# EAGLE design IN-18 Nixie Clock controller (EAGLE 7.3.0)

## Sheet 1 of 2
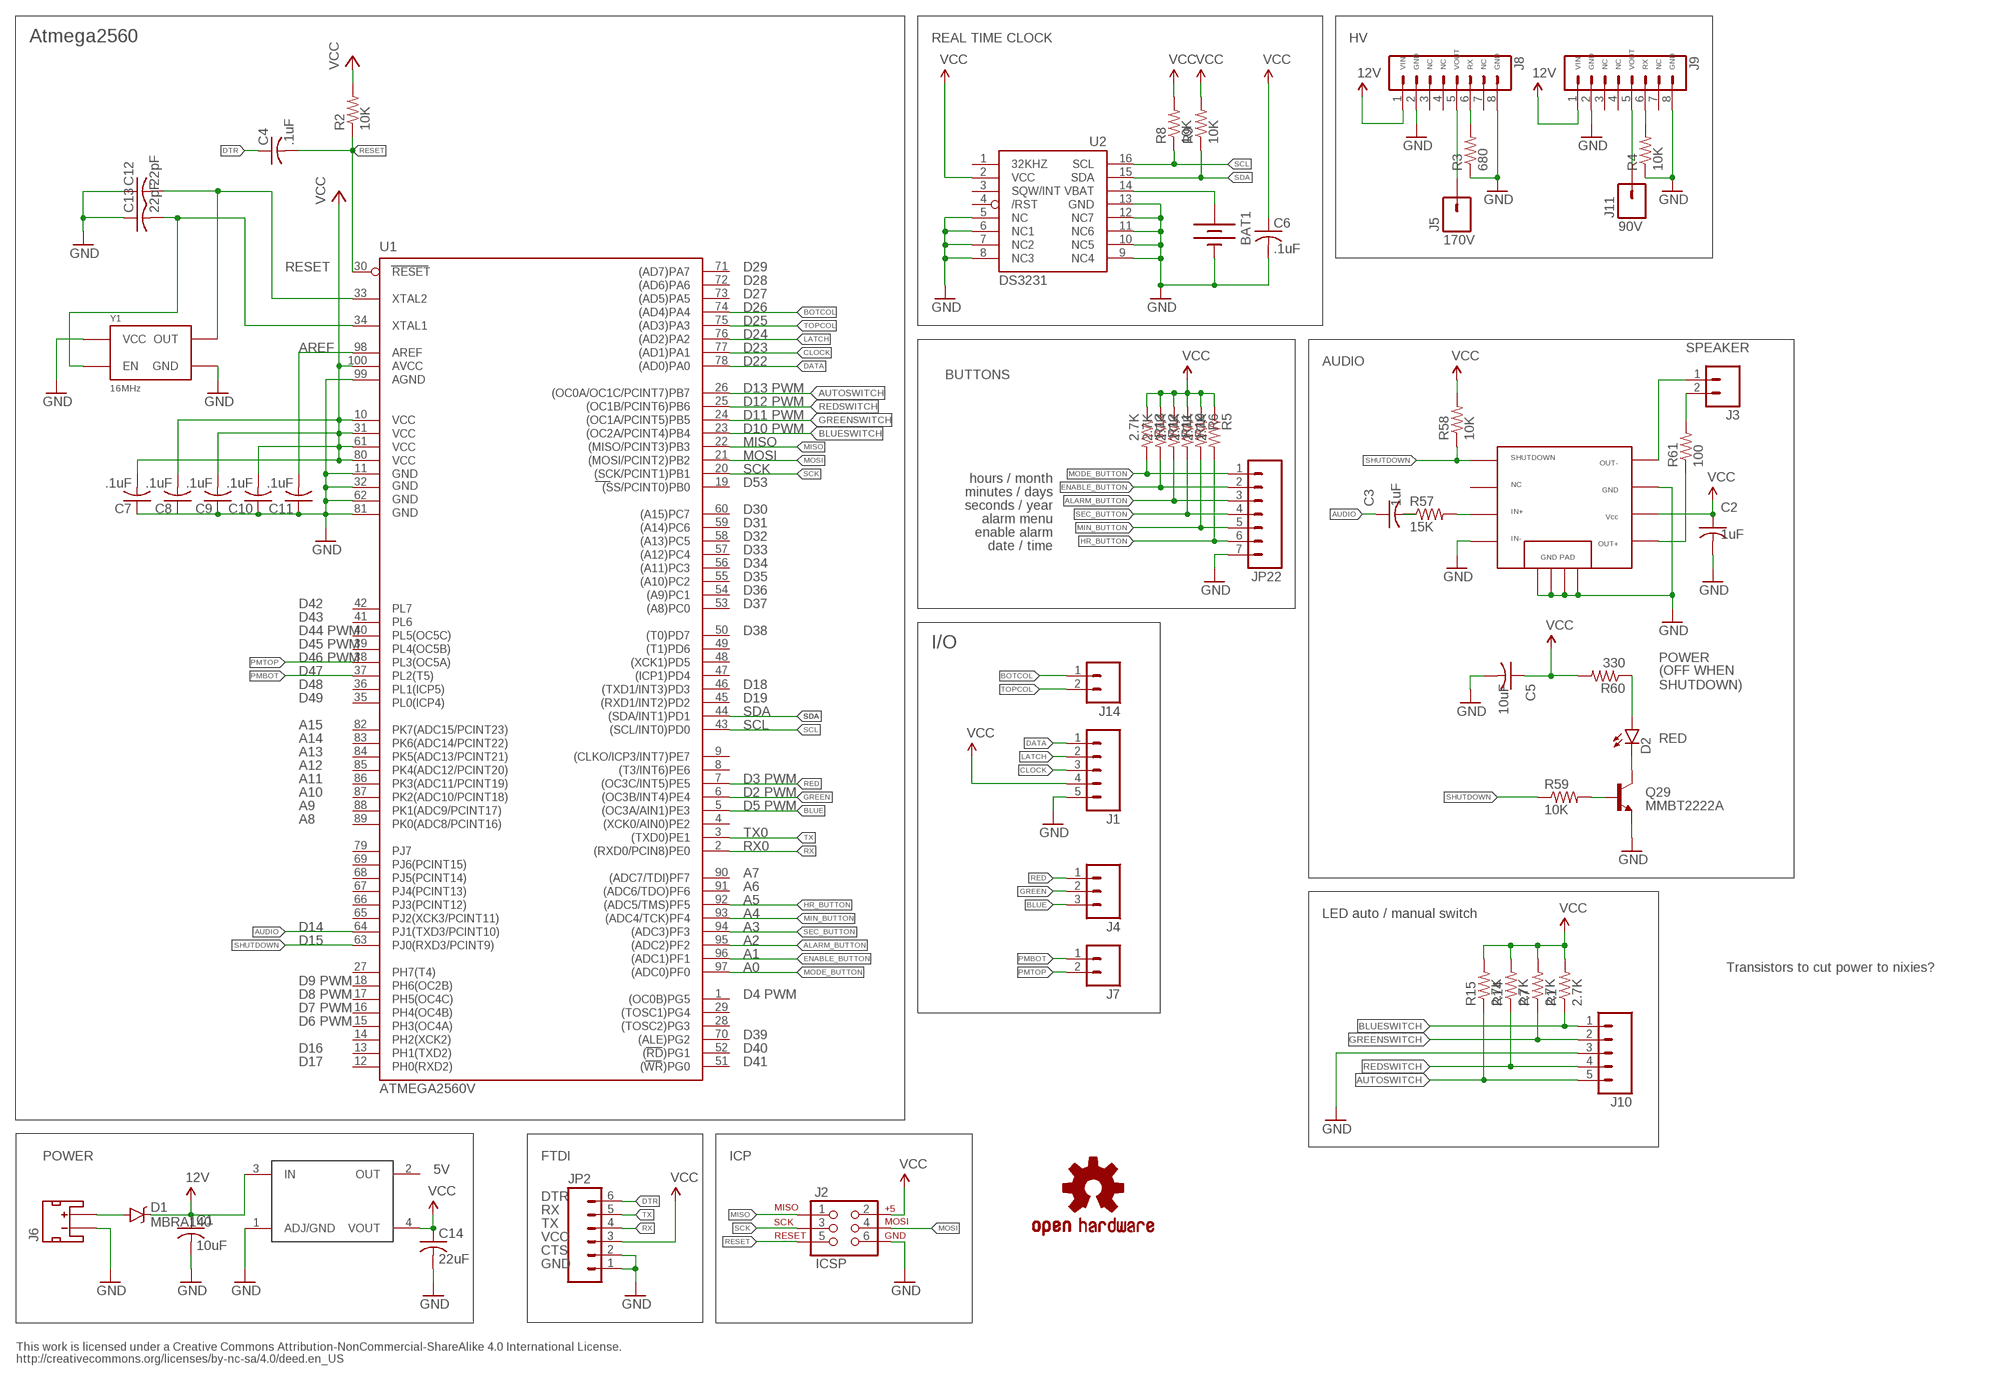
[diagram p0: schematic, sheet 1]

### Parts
BAT1  BATTERY12MM  [BATTCON_12MM]
C1  10uF  C-USC0805K  [C0805K]
C2  1uF  C-USC0805K  [C0805K]
C3  1uF  C-USC0805K  [C0805K]
C4  .1uF  C-USC0805K  [C0805K]
C5  10uF  C-USC0805K  [C0805K]
C6  .1uF  C-USC0805K  [C0805K]
C7  .1uF  C-USC0805K  [C0805K]
C8  .1uF  C-USC0805K  [C0805K]
C9  .1uF  C-USC0805K  [C0805K]
C10  .1uF  C-USC0805K  [C0805K]
C11  .1uF  C-USC0805K  [C0805K]
C12  22pF  C-USC0805K  [C0805K]
C13  22pF  C-USC0805K  [C0805K]
C14  22uF  C-USC0805K  [C0805K]
D1  MBRA140  [SMA-DIODE]
D2  LED0603  [LED-0603]
J1  M05PTH  [1X05]
J2  ICSP  AVR_SPI_PRG_6PTH  [2X3]
J3  M02PTH  [1X02]
J4  M03PTH  [1X03]
J5  M01SMDNS  [1X01NS]
J6  PWR  JST_2MM_MALE  [JST-2-SMD]
J7  M02PTH  [1X02]
J8  M08  [1X08_ROUND]
J9  M08  [1X08_ROUND]
J10  M05PTH  [1X05]
J11  M01SMDNS  [1X01NS]
J14  M02PTH  [1X02]
JP2  M06SILK_FEMALE_PTH  [1X06]
JP22  M07  [1X07]
LOGO1  OSHW-LOGOM  [OSHW-LOGO-M]
Q29  MMBT2222A  TRANSISTOR_NPNSOT23-3  [SOT23-3]
R1  2.7K  R-US_R0805  [R0805]
R2  10K  R-US_R0805  [R0805]
R3  680  R-US_R0805  [R0805]
R4  10K  R-US_R0805  [R0805]
R5  2.7K  R-US_R0805  [R0805]
R6  2.7K  R-US_R0805  [R0805]
R7  2.7K  R-US_R0805  [R0805]
R8  10K  R-US_R0805  [R0805]
R9  10K  R-US_R0805  [R0805]
R10  2.7K  R-US_R0805  [R0805]
R11  2.7K  R-US_R0805  [R0805]
R12  2.7K  R-US_R0805  [R0805]
R13  2.7K  R-US_R0805  [R0805]
R14  2.7K  R-US_R0805  [R0805]
R15  2.7K  R-US_R0805  [R0805]
R57  15K  R-US_R0805  [R0805]
R58  10K  R-US_R0805  [R0805]
R59  10K  R-US_R0805  [R0805]
R60  330  R-US_R0805  [R0805]
R61  100  R-US_R0805  [R0805]
U1  ATMEGA2560  ATMEGA2560AU  [TQFP100]
U2  DS3231  DS3231/SO  [SO16W]
U3  TPA2005  [MSOP8]
U4  LT1117  [LT1117]
Y1  16MHz  OSCILLATOR5X3  [CRYSTAL-SMD-5X3]

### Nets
12V: C1.1 D1.C J8.1 J9.1 U4.3(IN)
ALARM_BUTTON: JP22.3 R11.2 U1.95((ADC2)PF2)
AREF: C11.2 U1.98(AREF)
AUDIO: C3.1 U1.64(PJ1(TXD3/PCINT10))
AUTOSWITCH: J10.5 R15.1 U1.26((OC0A/OC1C/PCINT7)PB7)
BLUE: J4.3 U1.5((OC3A/AIN1)PE3)
BLUESWITCH: J10.1 R1.1 U1.23((OC2A/PCINT4)PB4)
BOTCOL: J14.1 U1.74((AD4)PA4)
CLOCK: J1.3 U1.77((AD1)PA1)
DATA: J1.1 U1.78((AD0)PA0)
DTR: C4.1 JP2.6
ENABLE_BUTTON: JP22.2 R12.2 U1.96((ADC1)PF1)
GND: BAT1.GND(-) C1.2 C2.2 C5.2 C6.2 C7.1 C8.1 C9.1 C10.1 C11.1 C12.1 C13.1 C14.2 J1.5 J2.6 J6.1(-) J8.2 J8.8 J9.2 J9.8 J10.3 JP2.1 JP2.2 JP22.7 Q29.2(E) R3.1 R4.1 U1.11(GND) U1.32(GND1) U1.62(GND2) U1.81(GND3) U1.99(AGND) U2.5(NC) U2.6(NC1) U2.7(NC2) U2.8(NC3) U2.9(NC4) U2.10(NC5) U2.11(NC6) U2.12(NC7) U2.13(GND) U3.4 U3.7 U3.A U3.B U3.C U3.D U4.1(ADJ/GND) Y1.2(GND) Y1.4(VCC)
GREEN: J4.2 U1.6((OC3B/INT4)PE4)
GREENSWITCH: J10.2 R7.1 U1.24((OC1A/PCINT5)PB5)
HR_BUTTON: JP22.6 R5.2 U1.92((ADC5/TMS)PF5)
IN+AMP: R57.2 U3.3
LATCH: J1.2 U1.76((AD2)PA2)
MIN_BUTTON: JP22.5 R6.2 U1.93((ADC4/TCK)PF4)
MISO: J2.1 U1.22((MISO/PCINT3)PB3)
MODE_BUTTON: JP22.1 R13.2 U1.97((ADC0)PF0)
MOSI: J2.4 U1.21((MOSI/PCINT2)PB2)
N$1: D1.A J6.2(+)
N$2: C12.2 U1.33(XTAL2) Y1.3(OUT)
N$3: C13.2 U1.34(XTAL1) Y1.1(EN)
N$6: J5.1 J8.5
N$7: J8.6 R3.2
N$11: J9.5 J11.1
N$12: J9.6 R4.2
N$15: BAT1.PWR@1(+) U2.14(VBAT)
N$28: J3.2 R61.2
N$29: D2.A R60.1
N$31: Q29.1(B) R59.2
N$33: D2.C Q29.3(C)
N$34: C3.2 R57.1
N$35: J3.1 U3.8
N$36: R61.1 U3.5
PMBOT: J7.1 U1.37(PL2(T5))
PMTOP: J7.2 U1.38(PL3(OC5A))
RED: J4.1 U1.7((OC3C/INT5)PE5)
REDSWITCH: J10.4 R14.1 U1.25((OC1B/PCINT6)PB6)
RESET: C4.2 J2.5 R2.1 U1.30(RESET)
RX: JP2.4 U1.2((RXD0/PCIN8)PE0)
SCK: J2.3 U1.20((SCK/PCINT1)PB1)
SCL: R8.1 U1.43((SCL/INT0)PD0) U2.16(SCL)
SDA: R9.1 U1.44((SDA/INT1)PD1) U2.15(SDA)
SEC_BUTTON: JP22.4 R10.2 U1.94((ADC3)PF3)
SHUTDOWN: R58.1 R59.1 U1.63(PJ0(RXD3/PCINT9)) U3.1
TOPCOL: J14.2 U1.75((AD3)PA3)
TX: JP2.5 U1.3((TXD0)PE1)
VCC: C2.1 C5.1 C6.1 C7.2 C8.2 C9.2 C10.2 C14.1 J1.4 J2.2 JP2.3 R1.2 R2.2 R5.1 R6.1 R7.2 R8.2 R9.2 R10.1 R11.1 R12.1 R13.1 R14.2 R15.2 R58.2 R60.2 U1.10(VCC) U1.31(VCC1) U1.61(VCC2) U1.80(VCC3) U1.100(AVCC) U2.2(VCC) U3.6 U4.4(VOUT)
Unconnected: J6.NC1(PAD1) J6.NC2(PAD2) J8.3 J8.4 J8.7 J9.3 J9.4 J9.7 U1.1((OC0B)PG5) U1.4((XCK0/AIN0)PE2) U1.8((T3/INT6)PE6) U1.9((CLKO/ICP3/INT7)PE7) U1.12(PH0(RXD2)) U1.13(PH1(TXD2)) U1.14(PH2(XCK2)) U1.15(PH3(OC4A)) U1.16(PH4(OC4B)) U1.17(PH5(OC4C)) U1.18(PH6(OC2B)) U1.19((SS/PCINT0)PB0) U1.27(PH7(T4)) U1.28((TOSC2)PG3) U1.29((TOSC1)PG4) U1.35(PL0(ICP4)) U1.36(PL1(ICP5)) U1.39(PL4(OC5B)) U1.40(PL5(OC5C)) U1.41(PL6) U1.42(PL7) U1.45((RXD1/INT2)PD2) U1.46((TXD1/INT3)PD3) U1.47((ICP1)PD4) U1.48((XCK1)PD5) U1.49((T1)PD6) U1.50((T0)PD7) U1.51((WR)PG0) U1.52((RD)PG1) U1.53((A8)PC0) U1.54((A9)PC1) U1.55((A10)PC2) U1.56((A11)PC3) U1.57((A12)PC4) U1.58((A13)PC5) U1.59((A14)PC6) U1.60((A15)PC7) U1.65(PJ2(XCK3/PCINT11)) U1.66(PJ3(PCINT12)) U1.67(PJ4(PCINT13)) U1.68(PJ5(PCINT14)) U1.69(PJ6(PCINT15)) U1.70((ALE)PG2) U1.71((AD7)PA7) U1.72((AD6)PA6) U1.73((AD5)PA5) U1.79(PJ7) U1.82(PK7(ADC15/PCINT23)) U1.83(PK6(ADC14/PCINT22)) U1.84(PK5(ADC13/PCINT21)) U1.85(PK4(ADC12/PCINT20)) U1.86(PK3(ADC11/PCINT19)) U1.87(PK2(ADC10/PCINT18)) U1.88(PK1(ADC9/PCINT17)) U1.89(PK0(ADC8/PCINT16)) U1.90((ADC7/TDI)PF7) U1.91((ADC6/TDO)PF6) U2.1(32KHZ) U2.3(SQW/INT) U2.4(/RST) U3.NC U4.2(OUT)

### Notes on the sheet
- Atmega2560 | REAL TIME CLOCK | HV
- VIN | GND | NC | NC | VOUT | RX | NC | GND | VIN | GND | NC | NC | VOUT | RX | NC | GND
- 90V
- 170V
- D29
- D28
- D27
- D26
- D25
- D24
- D23 | SPEAKER
- D22 | AUDIO
- BUTTONS
- D13 PWM
- D12 PWM
- D11 PWM
- D10 PWM
- MISO
- MOSI
- SCK | hours / month
- D53 | minutes / days
- seconds / year
- D30 | alarm menu
- D31 | enable alarm
- D32 | date / time
- D33
- D34
- D35
- D36
- D42 | D37
- D43
- D44 PWM | D38
- D45 PWM | I/O
- D46 PWM | POWER
- D47
- D48 | D18
- (OFF WHEN 
  SHUTDOWN)
- D49 | D19
- SDA
- A15 | SCL
- A14 | RED
- A13
- A12
- A11 | D3 PWM
- A10 | D2 PWM
- A9 | D5 PWM
- A8
- TX0
- RX0
- A7
- A6
- A5
- A4 | LED auto / manual switch
- D14 | A3
- D15 | A2
- A1
- A0 | Transistors to cut power to nixies?
- D9 PWM
- D8 PWM | D4 PWM
- D7 PWM
- D6 PWM
- D39
- D16 | D40
- D17 | D41
- ATMEGA2560V
- POWER | FTDI | ICP
- 5V
- DTR
- RX
- TX
- VCC
- CTS
- GND
- This work is licensed under a Creative Commons Attribution-NonCommercial-ShareAlike 4.0 International License.
  http://creativecommons.org/licenses/by-nc-sa/4.0/deed.en_US

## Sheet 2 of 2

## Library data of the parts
BAT1 = SparkFun-Electromechanical:BATTERY: Battery Holders; PROD_ID: BATT-08044
C1-C14 = adafruit:C-US: CAPACITOR, American symbol
D1 = SparkFun-DiscreteSemi:MBRA140: 40V, 1A Schottky rectifier; PROD_ID: DIO-08053
D2 = SparkFun-LED:LED: LEDs
J1 J10 = SparkFun-Connectors:M05: Header 5 Standard 5-pin 0.1" header. Use with straight break away headers (SKU : PRT-00116), right angle break away headers (PRT-00553), swiss pins (PRT-00743), machine pins (PRT-00117), and female headers (PRT-00115). Molex polarized connector foot print use with SKU : PRT-08230 with associated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
J2 = SparkFun:AVR_SPI_PRG_6: AVR ISP 6 Pin This is the reduced ISP connector for AVR programming. Common on Arduino. This footprint will take up less PCB space and can be used with a 10-pin to 6-pin adapter such as SKU: BOB-08508; OC_NEWARK: unknown
J3 J7 J14 = SparkFun-Connectors:M02: Standard 2-pin 0.1" header. Use with
J4 = SparkFun-Connectors:M03: Header 3 Standard 3-pin 0.1" header. Use with straight break away headers (SKU : PRT-00116), right angle break away headers (PRT-00553), swiss pins (PRT-00743), machine pins (PRT-00117), and female headers (PRT-00115). Molex polarized connector foot print use with SKU : PRT-08232 with associated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
J5 J11 = SparkFun-Connectors:M01: Header 1
J6 = SparkFun-Connectors:JST_2MM_MALE: Mates to single-cell LiPo batteries. CONN-11443 Now with smashable polarity marks!; BTM_NEG: -; BTM_POS: +; PROD_ID: CONN-11443; TOP_NEG: -; TOP_POS: +
J8 J9 = SparkFun-Connectors:M08: Header 8 Standard 8-pin 0.1" header. Use with straight break away headers (SKU : PRT-00116), right angle break away headers (PRT-00553), swiss pins (PRT-00743), machine pins (PRT-00117), and female headers (PRT-00115).; PROD_ID: CONN-08437
JP2 = SparkFun-Connectors:M06: Header 6 Standard 6-pin 0.1" header. Use with straight break away headers (SKU : PRT-00116), right angle break away headers (PRT-00553), swiss pins (PRT-00743), machine pins (PRT-00117), and female headers (PRT-00115). Molex polarized connector foot print use with SKU : PRT-08094 with associated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; PROD_ID: CONN-08437
JP22 = SparkFun-Connectors:M07: Header 7 Standard 7-pin 0.1" header. Use with straight break away headers (SKU : PRT-00116), right angle break away headers (PRT-00553), swiss pins (PRT-00743), machine pins (PRT-00117), and female headers (PRT-00115). NOTES ON THE VARIANTS LOCK and LOCK_LONGPADS... This footprint was designed to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
LOGO1 = SparkFun-Aesthetics:OSHW-LOGO: Open Source Hardware Logo
Q29 = SparkFun:TRANSISTOR_NPN: Transistor NPN BJT configuration in SOT23 package. MMBT2222 is the common NPN we use. Double check BCE configuration again layout.
R1-R15 R57-R61 = adafruit:R-US_: RESISTOR, American symbol
U1 = SparkFun:ATMEGA2560: MICROCONTROLLER 64/128/256 Kbytes FLASH 4 Kbytes EEPROM 8 Kbytes SRAM 86 General Purpose I/O pins 12-channels16-bit PWM 4 x Serial USARTs 16-channels 10-bit A/D; OC_NEWARK: unknown
U2 = adafruit:DS3231
U3 = TPA2005:TPA2005
U4 = LT1117:LT1117
Y1 = SparkFun-FreqCtrl:OSCILLATOR: Generic 5x3 and 7x5 oscillators

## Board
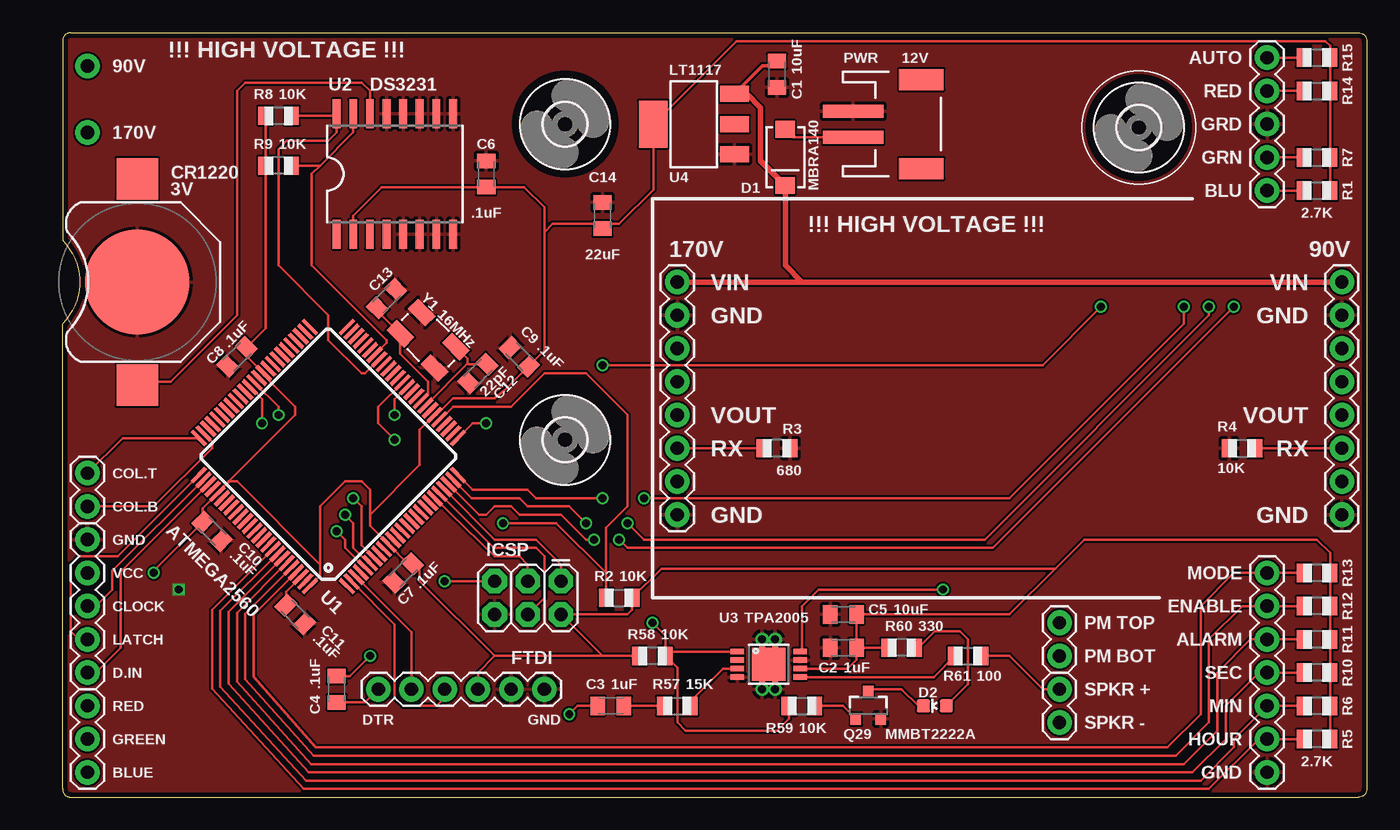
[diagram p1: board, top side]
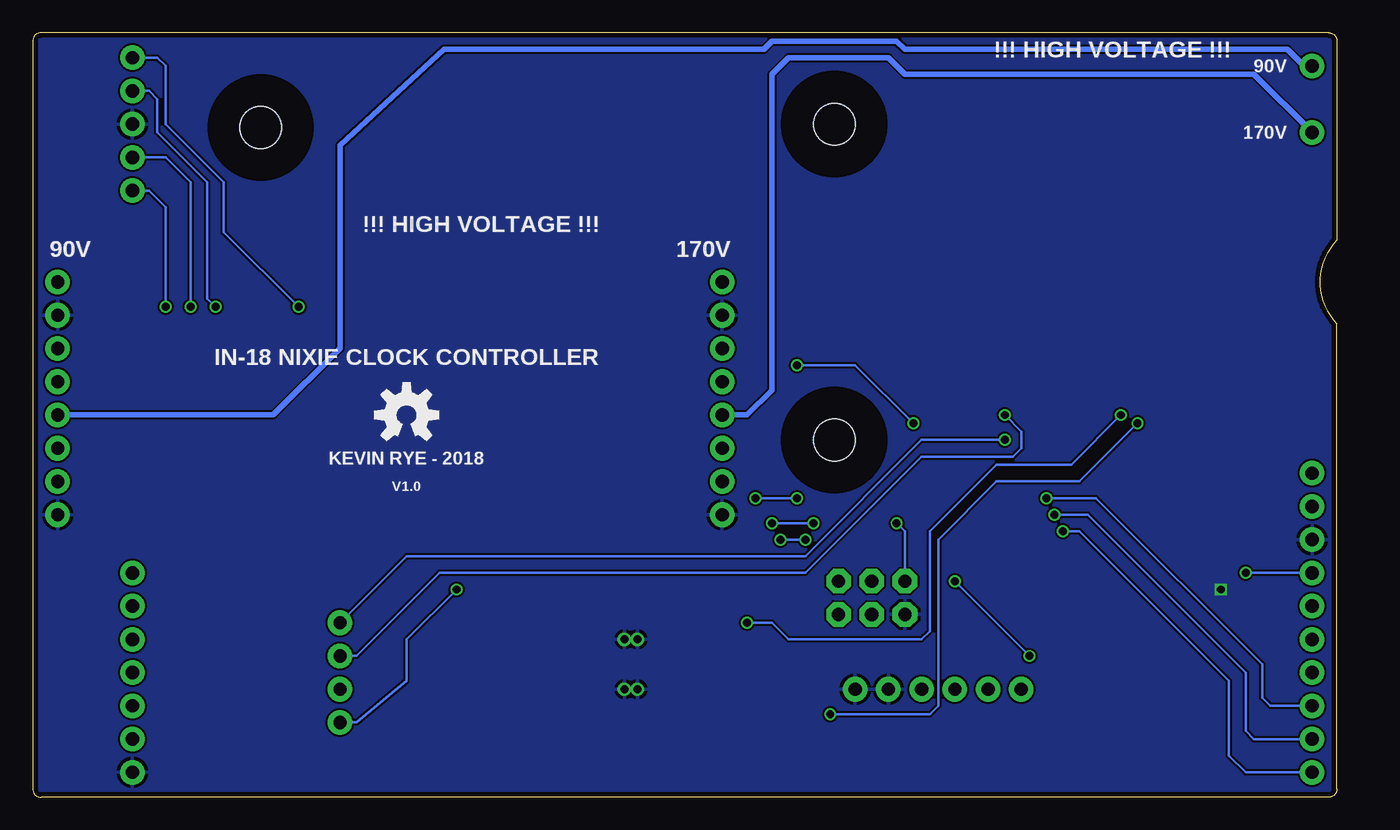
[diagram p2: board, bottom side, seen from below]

Size 99.7 x 58.42 mm. Coordinates in mm from the lower left corner, seen from the top.
Outline: 0.64,58.42 99.06,58.42 arc-90 99.7,57.79 99.7,0.64 arc-90 99.06,0 0.64,0 arc-90 0,0.64 0,36.2 arc90 0,42.55 0,57.79 arc-90 0.64,58.42
Copper layers (1*16): Top 0.035559375mm / dielectric 1.6mm / Bottom 0.035559375mm
Design rules "oshpark-2layer": minimum track width 6mil, minimum drill 10mil, track to track 6mil, track to pad 6mil, pad to pad 6mil, via to via 6mil, smd to smd 6mil, copper to edge 15mil, drill to drill 6mil, minimum pad ring 5mil, minimum via ring 5mil, stop-mask expansion 2.5mil, vias tented up to drill 0mil, thermal gap 10mil

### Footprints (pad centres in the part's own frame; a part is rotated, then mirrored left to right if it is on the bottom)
BATTCON_12MM = smd 8 x 8: GND 0,0 | smd 3.175 x 3.175: PWR@1 -7.874,0; PWR@2 7.874,0
C0805K = smd 1.1 x 1.4: 1 -1,0; 2 1,0
SMA-DIODE = smd 1.27 x 1.47: A -2.15,0; C 2.15,0
LED-0603 = smd 1 x 1: A 0,-0.877; C 0,0.877
1X05 = drill 1.016 pad 1.88: 1 0,0; 2 2.54,0; 3 5.08,0; 4 7.62,0; 5 10.16,0
2X3 = drill 1.016 pad 1.88 octagon: 1 0,0; 2 0,2.54; 3 2.54,0; 4 2.54,2.54; 5 5.08,0; 6 5.08,2.54
1X02 = drill 1.016 pad 1.88: 1 0,0; 2 2.54,0
1X03 = drill 1.016 pad 1.88: 1 0,0; 2 2.54,0; 3 5.08,0
1X01NS = drill 1.016 pad 1.88: 1 0,0
JST-2-SMD = smd 1 x 4.6: 1 -1,-3.7; 2 1,-3.7 | smd 1.6 x 3.4: NC1 -3.4,1.5; NC2 3.4,1.5
1X08_ROUND = drill 1.016 pad 1.88: 1 0,0; 2 2.54,0; 3 5.08,0; 4 7.62,0; 5 10.16,0; 6 12.7,0; 7 15.24,0; 8 17.78,0
1X06 = drill 1.016 pad 1.88: 1 0,0; 2 2.54,0; 3 5.08,0; 4 7.62,0; 5 10.16,0; 6 12.7,0
1X07 = drill 1.016 pad 1.88: 1 0,0; 2 2.54,0; 3 5.08,0; 4 7.62,0; 5 10.16,0; 6 12.7,0; 7 15.24,0
SOT23-3 = smd 0.8 x 0.9: 1 -0.95,-1; 2 0.95,-1; 3 0,1.1
R0805 = smd 1.1 x 1.4: 1 -1,0; 2 1,0
TQFP100 = smd 1.5 x 0.3: 1 -8,6; 2 -8,5.5; 3 -8,5; 4 -8,4.5; 5 -8,4; 6 -8,3.5; 7 -8,3; 8 -8,2.5; 9 -8,2; 10 -8,1.5; 11 -8,1; 12 -8,0.5; 13 -8,0; 14 -8,-0.5; 15 -8,-1; 16 -8,-1.5; 17 -8,-2; 18 -8,-2.5; 19 -8,-3; 20 -8,-3.5; 21 -8,-4; 22 -8,-4.5; 23 -8,-5; 24 -8,-5.5; 25 -8,-6; 51 8,-6; 52 8,-5.5; 53 8,-5; 54 8,-4.5; 55 8,-4; 56 8,-3.5; 57 8,-3; 58 8,-2.5; 59 8,-2; 60 8,-1.5; 61 8,-1; 62 8,-0.5; 63 8,0; 64 8,0.5; 65 8,1; 66 8,1.5; 67 8,2; 68 8,2.5; 69 8,3; 70 8,3.5; 71 8,4; 72 8,4.5; 73 8,5; 74 8,5.5; 75 8,6 | smd 0.3 x 1.5: 26 -6,-8; 27 -5.5,-8; 28 -5,-8; 29 -4.5,-8; 30 -4,-8; 31 -3.5,-8; 32 -3,-8; 33 -2.5,-8; 34 -2,-8; 35 -1.5,-8; 36 -1,-8; 37 -0.5,-8; 38 0,-8; 39 0.5,-8; 40 1,-8; 41 1.5,-8; 42 2,-8; 43 2.5,-8; 44 3,-8; 45 3.5,-8; 46 4,-8; 47 4.5,-8; 48 5,-8; 49 5.5,-8; 50 6,-8; 76 6,8; 77 5.5,8; 78 5,8; 79 4.5,8; 80 4,8; 81 3.5,8; 82 3,8; 83 2.5,8; 84 2,8; 85 1.5,8; 86 1,8; 87 0.5,8; 88 0,8; 89 -0.5,8; 90 -1,8; 91 -1.5,8; 92 -2,8; 93 -2.5,8; 94 -3,8; 95 -3.5,8; 96 -4,8; 97 -4.5,8; 98 -5,8; 99 -5.5,8; 100 -6,8
SO16W = smd 0.6 x 2.2: 1 -4.445,-4.6; 2 -3.175,-4.6; 3 -1.905,-4.6; 4 -0.635,-4.6; 5 0.635,-4.6; 6 1.905,-4.6; 7 3.175,-4.6; 8 4.445,-4.6; 9 4.445,4.6; 10 3.175,4.6; 11 1.905,4.6; 12 0.635,4.6; 13 -0.635,4.6; 14 -1.905,4.6; 15 -3.175,4.6; 16 -4.445,4.6
MSOP8 = smd 0.41 x 1.02: 1 -0.975,-2.4; 3 0.325,-2.4; 4 0.975,-2.4; 5 0.975,2.4; 6 0.325,2.4; 7 -0.325,2.4; 8 -0.975,2.4; NC -0.325,-2.4 | smd 1.02 x 0.41: 2 -1.13,0.5; 9 -1.13,-0.5; 10 1.13,-0.5; 11 1.13,0.5 | drill 0.61 pad 1.016: A -1.9,-0.5; B 1.91,-0.5; C 1.91,0.5; D -1.9,0.5 | smd 2.54 x 1.27: GND 0,0.635; GND1 0,0.635; GND* 0,-0.635
LT1117 = smd 1.219 x 2.235: 1 0.864,-1.194; 2 3.175,-1.194; 3 5.486,-1.194 | smd 3.6 x 2.2: 4 3.175,5.004
3,2 = hole 3.2: 0,0
CRYSTAL-SMD-5X3 = smd 1.9 x 1.1: 1 -1.85,-1.15; 2 1.85,-1.15; 3 1.85,1.15; 4 -1.85,1.15

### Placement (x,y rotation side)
BAT1  5.72,39.37 90 top
C1  54.61,55.25 270 top
C2  59.69,11.43 180 top
C3  41.91,6.99 0 top
C4  20.95,8.26 90 top
C5  59.69,13.97 180 top
C6  32.39,47.62 90 top
C7  26.04,17.14 45 top
C8  13.34,33.66 45 top
C9  34.93,33.66 315 top
C10  11.43,20.32 135 top
C11  17.78,13.97 135 top
C12  31.75,32.39 45 top
C13  24.77,38.1 225 top
C14  41.28,44.45 90 top
D1  55.25,48.9 270 top
D2  66.67,6.99 90 top
J1  1.91,9.53 90 top
J2  38.1,16.51 180 top
J3  76.2,5.71 90 top
J4  1.91,6.99 270 top
J5  1.91,50.8 270 top
J6  64.14,51.44 270 top
J7  76.2,10.79 90 top
J8  46.99,39.37 270 top
J9  97.79,39.37 270 top
J10  92.08,46.36 90 top
J11  1.91,55.88 270 top
J14  1.91,22.22 90 top
JP2  36.83,8.26 180 top
JP22  92.08,17.14 270 top
LOGO1  71.12,29.21 0 bottom
Q29  61.59,6.99 0 top
R1  95.89,46.36 0 top
R2  42.55,15.24 0 top
R3  54.61,26.67 180 top
R4  90.17,26.67 0 top
R5  95.89,4.45 180 top
R6  95.89,6.99 180 top
R7  95.89,48.9 0 top
R8  16.51,52.07 180 top
R9  16.51,48.26 180 top
R10  95.89,9.53 180 top
R11  95.89,12.06 180 top
R12  95.89,14.61 180 top
R13  95.89,17.14 180 top
R14  95.89,53.98 0 top
R15  95.89,56.52 0 top
R57  46.99,6.99 0 top
R58  45.09,10.79 180 top
R59  56.52,6.99 0 top
R60  64.14,11.43 180 top
R61  69.22,10.79 0 top
U1  20.32,26.04 135 top
U2  25.4,47.62 0 top
U3  53.98,10.16 270 top
U4  50.17,48.26 90 top
U$2  [3,2]  38.42,27.3 0 top
U$4  [3,2]  38.42,51.44 0 top
U$6  [3,2]  82.27,51.18 0 top
Y1  27.94,34.93 315 top

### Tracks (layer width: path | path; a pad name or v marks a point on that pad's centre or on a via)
12V
  Top 0.254: C1.1 54.61,55.88 53.49,55.88 U4.3 52.3,53.75
  Top 0.406: J9.1 56.52,39.37 | 56.52,39.37 J8.1 | 56.52,39.37 55.25,40.64 D1.C 53.34,48.65 53.34,52.71 52.3,53.75
ALARM_BUTTON
  Top 0.178: R11.2 JP22.3 90.81,12.06 88.27,9.53 88.27,5.08 85.73,2.54 18.99,2.54 13.34,8.83 13.34,14.1 U1.95
AREF
  Top 0.178: U1.98 17.07,15.72 C11.2
AUDIO  (via drill 0.61)
  Top 0.178: U1.64 15.24,30.41 v15.24,28.57 | v38.73,6.35 39.37,6.99 C3.1
  Bottom 0.178: v15.24,28.57 19.68,24.13 26.04,24.13 30.48,19.68 30.48,6.99 31.11,6.35 v38.73,6.35
AUTOSWITCH  (via drill 0.61)
  Top 0.178: R15.1 J10.5 | U1.26 31.35,28.57 v32.39,28.57 | v41.28,33.02 74.93,33.02 v79.38,37.47
  Bottom 0.178: v32.39,28.57 36.83,33.02 v41.28,33.02 | v79.38,37.47 85.09,43.18 85.09,46.99 89.53,51.44 89.53,55.88 90.17,56.52 J10.5
BLUE  (via drill 0.61)
  Top 0.178: U1.5 23.09,17.55 21.59,19.05 21.59,19.68 v20.95,20.32
  Bottom 0.178: v20.95,20.32 19.68,20.32 8.25,8.89 8.25,3.17 6.99,1.91 J4.3
BLUESWITCH  (via drill 0.61)
  Top 0.178: R1.1 J10.1 | U1.23 31.84,21.59 32.39,21.59 33.02,22.22 34.29,22.22 34.93,21.59 38.1,21.59 40.01,19.68 v40.64,19.68 | v42.55,19.68 43.18,19.05 71.12,19.05 v89.53,37.47
  Bottom 0.178: v40.64,19.68 v42.55,19.68 | v89.53,37.47 89.53,45.09 90.81,46.36 J10.1
BOTCOL
  Top 0.178: U1.74 11.43,27.15 11.43,26.67 6.99,22.22 J14.1
CLOCK
  Top 0.178: U1.77 3.81,17.3 3.81,15.88 2.54,14.61 J1.3
DATA
  Top 0.178: U1.78 4.45,17.23 4.45,11.43 2.54,9.53 J1.1
DTR
  Top 0.178: JP2.6 23.13,7.25 C4.1
ENABLE_BUTTON
  Top 0.178: JP22.2 R12.2 90.17,14.61 87.63,12.06 87.63,5.71 85.09,3.17 19.19,3.17 13.97,9.03 13.97,14.03 U1.96
GND  (via drill 0.61)
  other vias: 8.89,15.88
  pour Bottom: -0.63,59.05 100.33,59.05 100.33,-0.64 -0.63,-0.64
  pour Top: -1.27,59.05 100.97,59.69 100.97,-1.27 -1.27,-1.91
GREEN  (via drill 0.61)
  Top 0.178: U1.6 23.37,17.9 22.22,19.05 22.22,20.95 v21.59,21.59
  Bottom 0.178: v21.59,21.59 19.05,21.59 6.99,9.53 6.99,5.08 6.35,4.45 J4.2
GREENSWITCH  (via drill 0.61)
  Top 0.178: R7.1 J10.2 | U1.24 31.27,22.86 34.93,22.86 35.56,22.22 38.73,22.22 v40.01,20.95 | v43.18,20.95 44.45,19.68 70.48,19.68 87.63,36.83 v87.63,37.47
  Bottom 0.178: v40.01,20.95 v43.18,20.95 | v87.63,37.47 87.63,46.99 89.53,48.9 J10.2
HR_BUTTON
  Top 0.178: JP22.6 R5.2 91.44,4.45 87.63,0.64 18.44,0.64 11.43,8.28 11.43,14.32 U1.92
IN+AMP
  Top 0.178: U3.3 50.48,9.84 47.99,7.35 R57.2 48.26,7.25
LATCH
  Top 0.178: U1.76 4.21,18.41 1.27,18.41 0.64,17.78 0.64,12.7 1.27,12.06 J1.2
MIN_BUTTON
  Top 0.178: R6.2 JP22.5 89.53,4.45 89.53,3.81 87,1.27 18.61,1.27 12.07,8.45 12.07,14.24 U1.93
MISO
  Top 0.178: U1.22 33.03,19.68 36.2,19.68 38.1,17.78 J2.1
MODE_BUTTON
  Top 0.178: JP22.1 R13.2 89.53,17.14 87,14.61 87,6.35 84.45,3.81 19.36,3.81 14.61,9.2 14.61,13.96 U1.97
MOSI
  Top 0.178: U1.21 32.96,19.05 36.2,19.05 36.83,18.41 36.83,15.24 J2.4
N$1
  Top 0.178: J6.2 59.69,50.44 58.94,50.44 55.86,50.44 D1.A
N$2
  Top 0.178: Y1.3 30.98,33.52 30.98,33.16 | U1.33 30.98,33.16 | C12.2 31.04,33.09 30.98,33.16
N$3
  Top 0.178: C13.2 24.06,37.18 Y1.1 25.82,33.87 27.94,31.75 27.94,30.83 U1.34
N$6
  Bottom 0.406: J5.1 6.35,55.25 33.02,55.25 34.29,56.52 41.91,56.52 43.18,55.25 43.18,31.11 45.09,29.21 J8.5
N$7
  Top 0.178: J8.6 R3.2
N$11
  Bottom 0.406: J11.1 2.54,55.88 3.81,57.15 33.02,57.15 33.66,57.79 43.18,57.79 43.82,57.15 68.23,57.15 76.2,49.82 76.2,34.32 81.31,29.21 J9.5
N$12
  Top 0.178: J9.6 R4.2
N$15
  Top 0.178: U2.14 23.5,53.98 22.86,54.61 13.97,54.61 13.34,53.98 13.34,36.83 8.25,31.75 5.97,31.75 BAT1.PWR@1
N$28
  Top 0.178: R61.2 72.39,10.79 74.93,8.26 J3.2
N$29
  Top 0.178: D2.A 69.22,8.65 69.22,12.06 68.58,12.7 66.67,12.7 65.41,11.43 R60.1
N$31
  Top 0.178: Q29.1 59.65,6.99 R59.2
N$33
  Top 0.178: Q29.3 61.77,8.26 64.14,8.26 65.41,6.99 D2.C
N$34
  Top 0.178: C3.2 R57.1
N$35  (via drill 0.61)
  Top 0.178: v67.31,15.88 57.79,15.88 56.52,14.61 56.52,11.28 U3.8
  Bottom 0.178: v67.31,15.88 71.12,12.06 71.12,8.89 74.93,5.71 J3.1
N$36
  Top 0.178: R61.1 66.61,9.19 U3.5
PMBOT  (via drill 0.61)
  Top 0.178: U1.37 25.4,30.41 v25.4,29.21
  Bottom 0.178: v25.4,29.21 24.13,27.94 24.13,26.67 24.77,26.04 31.75,26.04 40.64,17.14 68.58,17.14 74.93,10.79 J7.1
PMTOP  (via drill 0.61)
  Top 0.178: U1.38 24.13,29.84 24.13,28.57 v25.4,27.3
  Bottom 0.178: v25.4,27.3 31.75,27.3 40.64,18.41 71.12,18.41 J7.2
RED  (via drill 0.61)
  Top 0.178: U1.7 22.86,19.25 22.86,22.22 v22.22,22.86
  Bottom 0.178: v22.22,22.86 18.41,22.86 5.72,10.16 5.72,7.62 5.08,6.99 J4.1
REDSWITCH  (via drill 0.61)
  Top 0.178: R14.1 J10.4 | U1.25 31.35,23.49 35.56,23.49 36.2,22.86 v41.28,22.86 | v44.45,22.86 72.39,22.86 85.73,36.2 v85.73,37.47
  Bottom 0.178: v41.28,22.86 v44.45,22.86 | v85.73,37.47 86.36,38.1 86.36,46.99 90.17,50.8 90.17,53.34 90.81,53.98 J10.4
RESET  (via drill 0.61)
  Top 0.178: U1.30 28.8,28.8 29.85,29.84 34.29,29.84 36.83,32.39 40.01,32.39 43.18,29.21 43.18,22.22 41.55,20.59 41.55,17.14 | J2.5 v29.21,16.51 | v23.5,10.79 21.95,9.26 C4.2 | 41.28,15.51 R2.1 41.55,17.14 | v33.66,20.95 37.73,20.95 41.55,17.14
  Bottom 0.178: J2.5 33.02,20.32 v33.66,20.95 | v29.21,16.51 v23.5,10.79
RX
  Top 0.178: U1.2 25.4,13.18 25.4,7.62 26.04,6.99 28.57,6.99 29.21,7.62 JP2.4
SCK
  Top 0.178: U1.20 33.02,18.41 34.93,18.41 35.56,17.78 J2.3
SCL
  Top 0.178: U2.16 20.8,52.07 | 20.8,52.07 R8.1 | 20.8,52.07 20.95,51.91 20.95,50.8 20.32,50.16 17.14,50.16 16.51,49.53 16.51,40.64 20.32,36.83 20.32,34.93 22.86,32.39 23.13,32.39 U1.43
SDA
  Top 0.178: U2.15 22.22,50.8 19.68,48.26 | 19.68,48.26 R9.1 | 19.68,48.26 19.05,47.62 19.05,40.64 24.77,34.93 24.77,34.72 U1.44
SEC_BUTTON
  Top 0.178: R10.2 JP22.4 91.44,9.53 88.9,6.99 88.9,4.45 86.36,1.91 18.81,1.91 12.7,8.65 12.7,14.17 U1.94
SHUTDOWN  (via drill 0.61)
  Top 0.178: R58.1 46.99,9.89 46.99,5.71 47.62,5.08 54.61,5.08 55.52,5.99 R59.1 | U3.1 46.43,11.13 arc90 R58.1 | U1.63 16.51,29.84 v16.51,29.21 | v45.09,13.34 46.09,12.34 R58.1
  Bottom 0.178: v16.51,29.21 20.32,25.4 26.04,25.4 31.11,20.32 31.11,12.7 31.75,12.06 41.91,12.06 43.18,13.34 v45.09,13.34
TOPCOL
  Top 0.178: U1.75 4.59,27.45 J14.2
TX
  Top 0.178: U1.3 26.67,12.61 JP2.5
VCC  (via drill 0.61)
  Top 0.178: U3.6 60,9.84 60.69,10.53 C2.1 | 60.69,11.16 C2.1 | R5.1 R6.1 R10.1 R11.1 R12.1 R13.1 96.89,18.68 95.89,19.68 78.11,19.68 75.88,17.46 | R60.2 C2.1 | C2.1 C5.1 72.39,13.97 75.88,17.46 | R58.2 41.28,10.79 | 41.28,10.79 33.02,10.79 | 33.02,10.79 31.75,9.53 JP2.3 | U1.80 10.72,22.09 C10.2 6.99,17.29 v6.99,17.14 | U2.2 22.22,44.45 24.4,46.62 C6.1 35.29,46.62 36.83,45.09 36.83,43.18 | R8.2 R9.2 15.51,35.83 C8.2 14.04,33.73 U1.61 15.37,32.26 17.78,29.84 17.78,29.21 12.7,24.13 | 12.7,24.13 12.7,24.07 U1.80 | U1.80 11.84,23.26 12.7,24.13 | 36.83,43.18 36.83,34.15 C9.2 33.8,31.11 33.02,30.48 29.85,30.48 28.58,29.22 U1.31 27.3,28.07 27.3,25.4 23.5,21.59 | U1.100 19.68,16.91 19.68,17.78 | 33.02,10.79 27.3,16.51 27.3,17.29 C7.2 26.38,17.85 U1.10 23.5,20.74 23.5,21.59 | 41.28,10.79 J2.2 43.18,13.97 43.55,14.34 R2.2 45.77,17.46 75.88,17.46 | 19.68,17.78 19.68,22.22 21.59,24.13 22.86,24.13 23.5,23.49 23.5,21.59 | 12.7,24.13 13.34,24.13 19.68,17.78 | 36.83,43.18 37.47,43.82 40.91,43.82 42.55,43.82 45.16,46.43 U4.4 51.51,57.79 96.52,57.79 96.89,57.42 R15.2 R14.2 R7.2 R1.2
  Top 0.254: C14.1 40.91,43.82
  Bottom 0.178: v6.99,17.14 J1.4

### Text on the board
Unrouted: This work is licensed under a Creative Commons Attribution-NonCommercial-ShareAlike 4.0 International License. / http://creativecommons.org/licenses/by-nc-sa/4.0/deed.en_US
tPlace: COL.T | COL.B | GND | VCC | CLOCK | LATCH | D.IN | RED | GREEN | BLUE
tNames: 90V | !!! HIGH VOLTAGE !!! | 12V | AUTO | RED | GRD | 170V | GRN | CR1220 | 3V | BLU | !!! HIGH VOLTAGE !!! | 170V | 90V | VIN | VIN | GND | GND | VOUT | VOUT | RX | RX | GND | GND | MODE | ENABLE | PM TOP | ALARM | FTDI | PM BOT | SEC | SPKR + | MIN | DTR | GND | SPKR - | HOUR | GND
bNames: 90V | !!! HIGH VOLTAGE !!! | 170V | !!! HIGH VOLTAGE !!! | 170V | 90V | IN-18 NIXIE CLOCK CONTROLLER | KEVIN RYE - 2018 | V1.0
